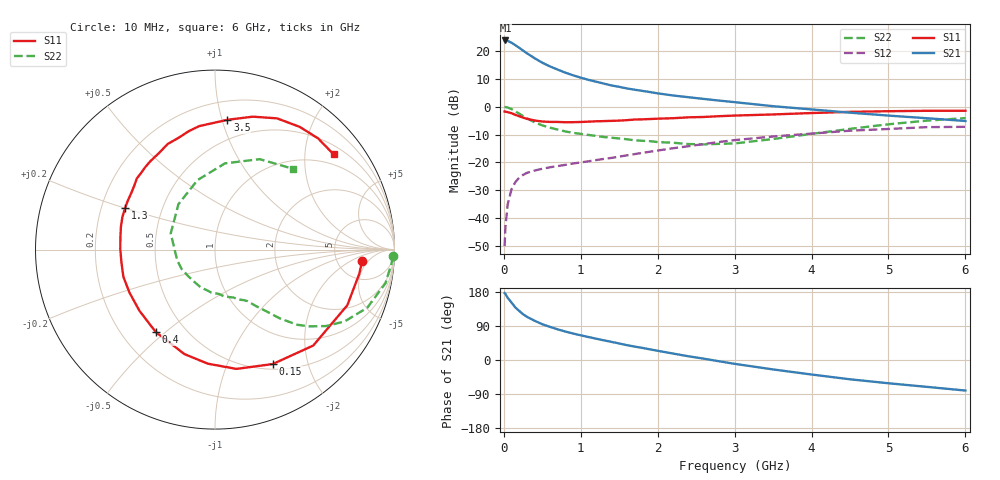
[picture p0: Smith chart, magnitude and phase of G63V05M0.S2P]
! SIEMENS Small Signal Semiconductors
! BFG193
! Si NPN RF Bipolar Junction Transistor in SOT223
! VCE = 3 V  IC = 5 mA
! Common Emitter S-Parameters:  August  1996
# GHz  S  MA  R  50
!  f  S11  S21  S12  S22
! GHz  MAG  ANG  MAG  ANG  MAG  ANG  MAG  ANG
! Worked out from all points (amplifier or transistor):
!   36 points, 10 MHz to 6 GHz, reference 50 ohm
!   highest |S21| = 23.8 dB at 20 MHz (marker M1)
!   |S21| within 3 dB of that: start of sweep to 217.9 MHz
!   unconditionally stable (mu >= 1): 1.104 GHz to 2.617 GHz
!   at 250 MHz: K = 0.34, MSG = 22.4 dB, |S12| = -24.5 dB
!   at 1.4 GHz: K = 1.09, MAG = 11.2 dB, |S12| = -18.4 dB
!   at 6 GHz: K = 0.89, MSG = 1.1 dB, |S12| = -7.2 dB
!   S11 on the Smith chart (normalised r, x): 10 MHz: 8.77, -3.56; 150 MHz: 0.57, -1.47; 400 MHz: 0.34, -0.46; 1.3 GHz: 0.30, +0.20; 3.5 GHz: 0.34, +1.04; 6 GHz: 0.71, +2.67
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0.01  0.8219 -4.6  15.53 176.7  0.0031 90.9  0.9912 -2.2
0.02  0.8152 -9.5  15.58 174.4  0.0066 86.3  0.9868 -4.5
0.05  0.7998 -22.8  15.26 164.1  0.0175 78.0  0.9679 -11.2
0.1  0.7651 -44.3  14.18 151.6  0.0328 69.5  0.9079 -20.9
0.15  0.7142 -63.2  12.78 138.5  0.0441 59.3  0.8257 -29.0
0.2  0.6754 -79.8  11.5 129.4  0.0531 53.8  0.7502 -34.6
0.25  0.6368 -93.6  10.23 120.8  0.0595 48.8  0.6766 -39.2
0.3  0.6066 -106.3  9.155 114.0  0.0645 45.7  0.6197 -42.5
0.4  0.5653 -125.8  7.462 103.6  0.0711 41.2  0.5243 -46.8
0.5  0.5417 -141.0  6.184 94.4  0.0766 38.7  0.4616 -49.5
0.6  0.5333 -153.4  5.316 87.4  0.0815 37.8  0.4205 -51.8
0.7  0.5325 -163.5  4.656 80.9  0.0856 37.3  0.3877 -54.1
0.9  0.5277 179.7  3.677 69.9  0.0954 37.4  0.3393 -57.8
1.1  0.5391 166.6  3.05 60.6  0.1043 38.2  0.3109 -63.6
1.3  0.5517 155.4  2.609 51.9  0.1151 38.3  0.2852 -69.2
1.6  0.5732 141.8  2.133 39.2  0.1336 37.5  0.2598 -80.8
2.2  0.6217 120.2  1.594 17.0  0.1791 32.4  0.2251 -110.6
2.8  0.6762 102.4  1.29 -3.4  0.2324 23.4  0.215 -150.2
3.5  0.7266 84.5  1.023 -24.9  0.2915 8.4  0.2626 160.0
4.5  0.8088 64.7  0.782 -50.9  0.3707 -12.1  0.3993 104.1
5.5  0.8449 47.2  0.621 -70.9  0.4293 -37.9  0.5622 63.7
6  0.8474 38.8  0.554 -80.6  0.435 -52.4  0.6245 46.2
